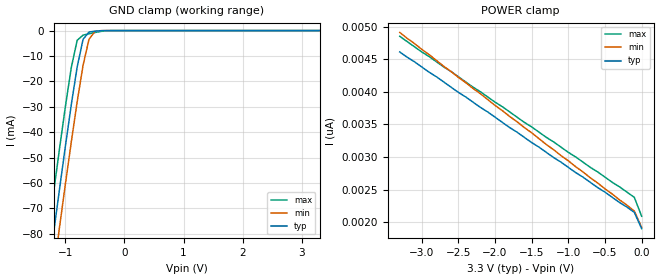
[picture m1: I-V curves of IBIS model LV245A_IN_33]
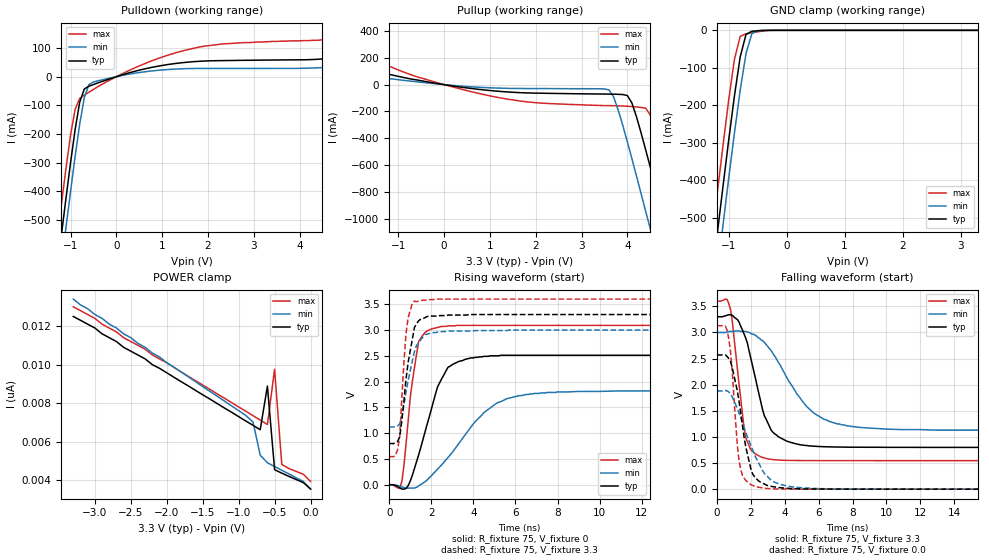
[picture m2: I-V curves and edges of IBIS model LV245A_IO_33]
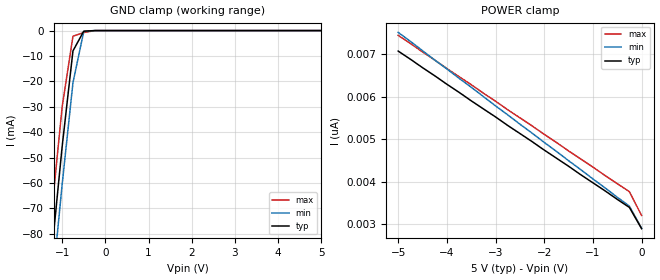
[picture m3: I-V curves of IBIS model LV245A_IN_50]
| TEXAS INSTRUMENTS INCORPORATED
| Standard Linear and Logic Group
| IBIS Model of SN74LV245A
| OCTAL BUS TRANSCEIVER WITH 3-STATE OUTPUTS
| SOIC 20-pin (DW), SOP 20-pin (NS), SSOP 20-pin (DB), TSSOP 20-pin (PW)
| and TVSOP 20-pin (DGV) Package
[IBIS Ver]   3.2
[Comment Char]  |_char
[File Name]   lv245a.ibs
[File Rev]   2.0 H_die
[Date]   May 29, 2000
[Source]   Data created from HSPICE simulations at TI-SLL.
[Notes]   The following is an IBIS list for the LV245A.
|   Please contact sllibis@ti.com with questions and
|   comments concerning SLL IBIS models.
|   The warning about non-monotonic V-I curves might be reported,
|   but it is nano ampere region and negligible.
|   The warning about AC Rising Endpoint might be reported,
|   but it is due to HSPICE issue and negligible.
[Disclaimer] Property of Texas Instruments Incorporated.  Unauthorized
   reproduction and/or distribution is strictly prohibited.
   This product is protected under copyright law.
   Created 2000, (C) Copyright 2000, Texas Instruments Inc.,
   All Rights Reserved.
   UNLESS THERE IS A SIGNED, WRITTEN AGREEMENT TO THE
   CONTRARY, TEXAS INSTRUMENTS () IS PROVIDING THE IBIS
   MODELS  AND WITHOUT ANY WARRANTY, EXPRESSED OR
   IMPLIED.  TI assumes no liability for:
   1) the accuracy of the IBIS models provided to your
   company;
   2) the proper functioning of these IBIS Models in your
   design or for any resulting applications; or
   3) infringement of patents, copyrights or intellectual
   property rights resulting from your use of these IBIS
   models.
   TI provides IBIS Models as a service to our customers.
   You and your company shall not distribute, sell or give
   these models to anyone else without prior written
   permission from TI.
   TI reserves the right to make changes to our products or
   to discontinue any semiconductor product or service
   without notice, and advises our customers to obtain the
   latest version of relevant information to verify, before
   placing orders, that the information being relied on is
   current.
   Please be aware that your receipt and use of the IBIS
   information provided shall serve as acceptance of these
   terms and conditions.  If you do not accept these terms,
   you should return or destroy the IBIS models and any
   other accompanying information immediately.
|   Component LV245A_DW
[Component]   LV245A_DW
[Manufacturer]  Texas Instruments, Inc.
[Package]
|   typ   min   max
R_pkg   0.038   0.033   0.045
L_pkg   5.012nH   4.110nH   6.349nH
C_pkg   0.717pF   0.530pF   0.868pF
[Pin]   signal_name   model_name   R_pin   L_pin   C_pin
1   DIR   LV245A_IN   0.042   6.336nH   0.865pF
2   A1   LV245A_IO   0.043   5.542nH   0.867pF
3   A2   LV245A_IO   0.034   4.714nH   0.732pF
4   A3   LV245A_IO   0.034   4.377nH   0.591pF
5   A4   LV245A_IO   0.036   4.130nH   0.533pF
6   A5   LV245A_IO   0.035   4.111nH   0.530pF
7   A6   LV245A_IO   0.034   4.284nH   0.583pF
8   A7   LV245A_IO   0.034   4.634nH   0.726pF
9   A8   LV245A_IO   0.040   5.518nH   0.865pF
10   GND   GND   0.043   6.349nH   0.866pF
11   B8   LV245A_IO   0.041   6.281nH   0.861pF
12   B7   LV245A_IO   0.045   5.561nH   0.868pF
13   B6   LV245A_IO   0.033   4.778nH   0.742pF
14   B5   LV245A_IO   0.035   4.414nH   0.596pF
15   B4   LV245A_IO   0.035   4.110nH   0.533pF
16   B3   LV245A_IO   0.036   4.130nH   0.533pF
17   B2   LV245A_IO   0.034   4.377nH   0.591pF
18   B1   LV245A_IO   0.034   4.714nH   0.731pF
19   OE_NOT   LV245A_IN   0.043   5.569nH   0.868pF
20   VCC   POWER   0.042   6.308nH   0.864pF
|   Component LV245A_NS
[Component]   LV245A_NS
[Manufacturer]  Texas Instruments, Inc.
[Package]
|   typ   min   max
R_pkg   0.044   0.029   0.058
L_pkg   3.666nH   2.317nH   5.115nH
C_pkg   0.548pF   0.316pF   0.725pF
[Pin]   signal_name   model_name   R_pin   L_pin   C_pin
1   DIR   LV245A_IN   0.058   5.115nH   0.725pF
2   A1   LV245A_IO   0.053   4.591nH   0.724pF
3   A2   LV245A_IO   0.049   3.754nH   0.572pF
4   A3   LV245A_IO   0.029   2.549nH   0.388pF
5   A4   LV245A_IO   0.031   2.317nH   0.316pF
6   A5   LV245A_IO   0.031   2.317nH   0.316pF
7   A6   LV245A_IO   0.029   2.556nH   0.399pF
8   A7   LV245A_IO   0.049   3.754nH   0.579pF
9   A8   LV245A_IO   0.053   4.591nH   0.724pF
10   GND   GND   0.058   5.115nH   0.725pF
11   B8   LV245A_IO   0.058   5.115nH   0.725pF
12   B7   LV245A_IO   0.053   4.591nH   0.724pF
13   B6   LV245A_IO   0.049   3.754nH   0.579pF
14   B5   LV245A_IO   0.029   2.557nH   0.399pF
15   B4   LV245A_IO   0.031   2.317nH   0.316pF
16   B3   LV245A_IO   0.031   2.317nH   0.316pF
17   B2   LV245A_IO   0.029   2.557nH   0.399pF
18   B1   LV245A_IO   0.049   3.754nH   0.579pF
19   OE_NOT   LV245A_IN   0.053   4.591nH   0.724pF
20   VCC   POWER   0.058   5.115nH   0.725pF
|   Component LV245A_DB
[Component]   LV245A_DB
[Manufacturer]  Texas Instruments, Inc.
[Package]
|   typ   min   max
R_pkg   0.040   0.035   0.051
L_pkg   3.495nH   3.035nH   4.314nH
C_pkg   0.420pF   0.346pF   0.502pF
[Pin]   signal_name   model_name   R_pin   L_pin   C_pin
1   DIR   LV245A_IN   0.049   4.310nH   0.502pF
2   A1   LV245A_IO   0.048   3.903nH   0.487pF
3   A2   LV245A_IO   0.035   3.189nH   0.396pF
4   A3   LV245A_IO   0.035   3.036nH   0.347pF
5   A4   LV245A_IO   0.035   3.035nH   0.367pF
6   A5   LV245A_IO   0.035   3.035nH   0.367pF
7   A6   LV245A_IO   0.035   3.036nH   0.347pF
8   A7   LV245A_IO   0.035   3.189nH   0.397pF
9   A8   LV245A_IO   0.047   3.899nH   0.488pF
10   GND   GND   0.051   4.314nH   0.500pF
11   B8   LV245A_IO   0.051   4.314nH   0.500pF
12   B7   LV245A_IO   0.047   3.899nH   0.488pF
13   B6   LV245A_IO   0.035   3.189nH   0.397pF
14   B5   LV245A_IO   0.035   3.036nH   0.346pF
15   B4   LV245A_IO   0.035   3.035nH   0.367pF
16   B3   LV245A_IO   0.035   3.035nH   0.367pF
17   B2   LV245A_IO   0.035   3.036nH   0.346pF
18   B1   LV245A_IO   0.035   3.189nH   0.397pF
19   OE_NOT   LV245A_IN   0.047   3.899nH   0.488pF
20   VCC   POWER   0.051   4.314nH   0.502pF
|   Component LV245A_PW
[Component]   LV245A_PW
[Manufacturer]  Texas Instruments, Inc.
[Package]
|   typ   min   max
R_pkg   0.035   0.024   0.047
L_pkg   2.399nH   1.710nH   3.250nH
C_pkg   0.284pF   0.166pF   0.418pF
[Pin]   signal_name   model_name   R_pin   L_pin   C_pin
1   DIR   LV245A_IN   0.041   3.102nH   0.410pF
2   A1   LV245A_IO   0.040   2.777nH   0.363pF
3   A2   LV245A_IO   0.029   2.194nH   0.260pF
4   A3   LV245A_IO   0.025   1.710nH   0.166pF
5   A4   LV245A_IO   0.025   1.740nH   0.191pF
6   A5   LV245A_IO   0.024   1.763nH   0.193pF
7   A6   LV245A_IO   0.024   1.817nH   0.174pF
8   A7   LV245A_IO   0.028   2.256nH   0.265pF
9   A8   LV245A_IO   0.045   2.887nH   0.368pF
10   GND   GND   0.047   3.250nH   0.417pF
11   B8   LV245A_IO   0.046   3.244nH   0.418pF
12   B7   LV245A_IO   0.046   2.961nH   0.375pF
13   B6   LV245A_IO   0.033   2.334nH   0.268pF
14   B5   LV245A_IO   0.029   1.915nH   0.179pF
15   B4   LV245A_IO   0.031   1.934nH   0.203pF
16   B3   LV245A_IO   0.032   1.917nH   0.201pF
17   B2   LV245A_IO   0.030   1.833nH   0.173pF
18   B1   LV245A_IO   0.036   2.324nH   0.268pF
19   OE_NOT   LV245A_IN   0.042   2.869nH   0.372pF
20   VCC   POWER   0.042   3.160nH   0.414pF
|   Component LV245A_DGV
[Component]   LV245A_DGV
[Manufacturer]  Texas Instruments, Inc.
[Package]
|   typ   min   max
R_pkg   0.044   0.038   0.048
L_pkg   2.561nH   2.236nH   2.961nH
C_pkg   0.342pF   0.264pF   0.446pF
[Pin]   signal_name   model_name   R_pin   L_pin   C_pin
1   DIR   LV245A_IN   0.044   2.935nH   0.417pF
2   A1   LV245A_IO   0.042   2.869nH   0.446pF
3   A2   LV245A_IO   0.043   2.399nH   0.316pF
4   A3   LV245A_IO   0.044   2.236nH   0.265pF
5   A4   LV245A_IO   0.046   2.278nH   0.264pF
6   A5   LV245A_IO   0.045   2.274nH   0.264pF
7   A6   LV245A_IO   0.044   2.285nH   0.269pF
8   A7   LV245A_IO   0.043   2.452nH   0.320pF
9   A8   LV245A_IO   0.044   2.900nH   0.446pF
10   GND   GND   0.044   2.961nH   0.418pF
11   B8   LV245A_IO   0.045   2.954nH   0.418pF
12   B7   LV245A_IO   0.042   2.847nH   0.443pF
13   B6   LV245A_IO   0.045   2.453nH   0.319pF
14   B5   LV245A_IO   0.045   2.297nH   0.269pF
15   B4   LV245A_IO   0.048   2.334nH   0.268pF
16   B3   LV245A_IO   0.048   2.335nH   0.267pF
17   B2   LV245A_IO   0.046   2.299nH   0.268pF
18   B1   LV245A_IO   0.046   2.457nH   0.320pF
19   OE_NOT   LV245A_IN   0.043   2.848nH   0.441pF
20   VCC   POWER   0.038   2.812nH   0.408pF
[Model Selector]   LV245A_IN
LV245A_IN_33   3.3-V Vcc Input Model
LV245A_IN_50   5.0-V Vcc Input Model
[Model Selector]   LV245A_IO
LV245A_IO_33   3.3-V Vcc Output Model
LV245A_IO_50   5.0-V Vcc Output Model
| Models and submodels in the file (4): LV245A_IN_33 (Input), LV245A_IO_33 (I/O), LV245A_IN_50 (Input), LV245A_IO_50 (I/O)
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|   Model LV245A_IN_33
[Model]   LV245A_IN_33
Model_type  Input
Polarity   Inverting
Vinl = 0.99
Vinh = 2.31
| variable   typ   min   max
C_comp   1.30pf   0.98pf   1.62pf
[Temperature Range]   25   85   -40
[Voltage Range]   3.3   3.0   3.6
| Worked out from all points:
|   GND clamp passes 1 mA (typ) near -0.61 V on its own axis
[GND Clamp]
|   Voltage   I(typ)   I(min)   I(max)
-3.3V     -460mA     -475mA     -445mA
-1.3V     -97.5mA    -113mA     -81.5mA
-1.2V     -79.9mA    -95mA      -63.9mA
-1.1V     -62.6mA    -77.6mA    -46.7mA
-1V       -45.6mA    -60.5mA    -30mA
-900mV    -29.2mA    -43.9mA    -14.6mA
-800mV    -14.3mA    -28mA      -3.81mA
-700mV    -3.42mA    -13.6mA    -1.78mA
-600mV    -581uA     -3.4mA     -1.25mA
-500mV    -233uA     -353uA     -759uA
-400mV    -58.1uA    -21.9uA    -324uA
3.3V      1.9nA      2.34nA     1.69nA
[POWER Clamp]
|   Voltage   I(typ)   I(min)   I(max)
-3.3V     4.61nA     4.91nA     4.85nA
-3V       4.38nA     4.65nA     4.61nA
-100mV    2.15nA     2.17nA     2.38nA
0V        1.9nA      1.92nA     2.09nA
|   Model LV245A_IO_33
[Model]   LV245A_IO_33
Model_type  I/O
Polarity   Non-Inverting
Enable   Active-Low
Vinl = 0.99
Vinh = 2.31
Vmeas = 1.65v
Cref = 15pf
| variable   typ   min   max
C_comp   6.0pf   4.5pf   7.5pf
[Temperature Range]   25   85   -40
[Voltage Range]   3.3   3.0   3.6
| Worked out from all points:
|   slope of the pulldown table from 0 to 0.495 V, typ, clamps not added: 21.9 ohm
|   slope of the pullup table from 0 to 0.495 V, typ, clamps not added: 20.4 ohm
|   GND clamp passes 1 mA (typ) near -0.48 V on its own axis
|   rising waveform, R_fixture 75, V_fixture 0: 20-80 % time 1.09ns typ, 2.25ns min, 519ps max; typ from 0 V to 2.51 V
|   falling waveform, R_fixture 75, V_fixture 3.3: 20-80 % time 1.17ns typ, 2.33ns min, 629ps max; typ from 3.3 V to 0.8 V
|   rising waveform, R_fixture 75, V_fixture 3.3: 20-80 % time 476ps typ, 557ps min, 289ps max; typ from 0.8 V to 3.3 V
|   falling waveform, R_fixture 75, V_fixture 0.0: 20-80 % time 827ps typ, 1.41ns min, 439ps max; typ from 2.57 V to 0 V
[Pulldown]
|   Voltage   I(typ)   I(min)   I(max)
-3.3V     -3.39A     -3.48A     -3.29A
-1.3V     -682mA     -784mA     -575mA
-1.2V     -552mA     -654mA     -445mA
-1.1V     -424mA     -526mA     -320mA
-900mV    -184mA     -278mA     -114mA
-800mV    -88.6mA    -165mA     -75.6mA
-700mV    -43mA      -73.3mA    -64.1mA
-600mV    -33.3mA    -27.7mA    -54.3mA
-500mV    -27.3mA    -18.4mA    -44.3mA
700mV     30.1mA     18.7mA     50.8mA
1.9V      54.5mA     28.8mA     106mA
6.6V      77.4mA     36.3mA     168mA
[Pullup]
|   Voltage   I(typ)   I(min)   I(max)
-3.3V     226mA      126mA      420mA
-700mV    40.5mA     25.1mA     70.6mA
600mV     -28.8mA    -16.4mA    -52.8mA
3.6V      -70.5mA    -39.7mA    -156mA
3.8V      -72.1mA    -188mA     -158mA
4.1V      -136mA     -551mA     -163mA
4.4V      -484mA     -942mA     -175mA
4.5V      -612mA     -1.07A     -225mA
4.8V      -1.01A     -1.48A     -581mA
5.1V      -1.41A     -1.88A     -977mA
5.2V      -1.54A     -2.02A     -1.11A
6.6V      -3.45A     -3.92A     -3.02A
[GND Clamp]
|   Voltage   I(typ)   I(min)   I(max)
-3.3V     -3.39A     -3.48A     -3.29A
-1.3V     -680mA     -783mA     -571mA
-1.2V     -549mA     -652mA     -440mA
-1.1V     -421mA     -524mA     -312mA
-1V       -295mA     -397mA     -188mA
-900mV    -176mA     -275mA     -78mA
-800mV    -71.1mA    -160mA     -16.2mA
-700mV    -11.1mA    -62.3mA    -9.19mA
-600mV    -2.57mA    -9.26mA    -6.5mA
-500mV    -1.21mA    -785uA     -4.03mA
-200mV    -3.4nA     -86.6nA    -8.11uA
3.3V      3.56nA     4.34nA     3.34nA
[POWER Clamp]
|   Voltage   I(typ)   I(min)   I(max)
-3.3V     12.5nA     13.4nA     13nA
-3V       11.9nA     12.6nA     12.4nA
-2.6V     10.9nA     11.6nA     11.4nA
-2.3V     10.3nA     10.9nA     10.8nA
-900mV    7.08nA     7.37nA     7.59nA
-800mV    6.86nA     7.03nA     7.36nA
-700mV    6.63nA     5.31nA     7.13nA
-600mV    8.89nA     4.92nA     6.9nA
-500mV    4.56nA     4.72nA     9.76nA
-400mV    4.38nA     4.53nA     4.83nA
-100mV    3.89nA     3.95nA     4.32nA
0V        3.56nA     3.55nA     3.95nA
[Ramp]
| variable   typ   min   max
dV/dt_r   1.51E+00/1.07E-09   1.10E+00/2.25E-09   1.86E+00/5.05E-10
dV/dt_f   1.52E+00/1.14E-09   1.14E+00/2.30E-09   1.86E+00/5.93E-10
R_load = 75
[Rising Waveform]
R_fixture = 75
V_fixture = 0
|   Time   V(typ)   V(min)   V(max)
0s        0V         0V         0V
600ps     -82.7mV    -43mV      60.9mV
1ns       71.3mV     -64.9mV    1.69V
1.4ns     581mV      -22.7mV    2.78V
2ns       1.46V      174mV      3.02V
2.3ns     1.9V       304mV      3.05V
3ns       2.33V      628mV      3.08V
4.5ns     2.49V      1.4V       3.09V
6.2ns     2.51V      1.73V      3.09V
25ns      2.51V      1.82V      3.09V
[Falling Waveform]
R_fixture = 75
V_fixture = 3.3
V_fixture_min = 3.0
V_fixture_max = 3.6
|   Time   V(typ)   V(min)   V(max)
0s        3.3V       3V         3.6V
800ps     3.34V      3.02V      3.44V
1.3ns     3.2V       3.03V      2.02V
1.7ns     2.89V      3.02V      985mV
2.7ns     1.51V      2.84V      605mV
3.2ns     1.13V      2.65V      571mV
4.1ns     922mV      2.15V      552mV
5.6ns     825mV      1.49V      548mV
7.1ns     807mV      1.25V      547mV
25ns      800mV      1.12V      546mV
[Rising Waveform]
R_fixture = 75
V_fixture = 3.3
V_fixture_min = 3.0
V_fixture_max = 3.6
|   Time   V(typ)   V(min)   V(max)
0s        800mV      1.12V      546mV
400ps     838mV      1.14V      678mV
500ps     931mV      1.18V      933mV
700ps     1.63V      1.54V      2.38V
800ps     2.05V      1.8V       2.93V
900ps     2.37V      2.02V      3.24V
1.2ns     3.05V      2.58V      3.56V
1.7ns     3.24V      2.91V      3.58V
2.8ns     3.29V      2.98V      3.6V
25ns      3.3V       3V         3.6V
[Falling Waveform]
R_fixture = 75
V_fixture = 0.0
|   Time   V(typ)   V(min)   V(max)
0s        2.57V      1.88V      3.13V
600ps     2.54V      1.88V      3.04V
800ps     2.44V      1.82V      2.63V
1.2ns     1.88V      1.55V      848mV
1.3ns     1.69V      1.46V      546mV
1.7ns     808mV      1.09V      167mV
2.1ns     293mV      755mV      71.5mV
3.2ns     53.4mV     170mV      8.62mV
4.7ns     7.75mV     35.6mV     1.8mV
25ns      31.2uV     73.7uV     16.5uV
|   Model LV245A_IN_50
[Model]   LV245A_IN_50
Model_type  Input
Polarity   Inverting
Vinl = 1.5
Vinh = 3.5
| variable   typ   min   max
C_comp   1.30pf   0.98pf   1.62pf
[Temperature Range]   25   85   -40
[Voltage Range]   5.0   4.5   5.5
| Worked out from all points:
|   GND clamp passes 1 mA (typ) near -0.52 V on its own axis
[GND Clamp]
|   Voltage   I(typ)   I(min)   I(max)
-5V       -773mA     -786mA     -758mA
-1.5V     -133mA     -148mA     -117mA
-1.25V    -88.7mA    -104mA     -72.7mA
-1V       -45.6mA    -60.5mA    -30mA
-750mV    -7.99mA    -20.5mA    -2.23mA
-500mV    -233uA     -353uA     -759uA
-250mV    -2.63nA    -182nA     -26.9uA
5V        2.9nA      3.64nA     2.54nA
[POWER Clamp]
|   Voltage   I(typ)   I(min)   I(max)
-5V       7.08nA     7.52nA     7.45nA
-1.5V     4.37nA     4.5nA      4.73nA
-250mV    3.4nA      3.43nA     3.77nA
0V        2.9nA      2.91nA     3.21nA
